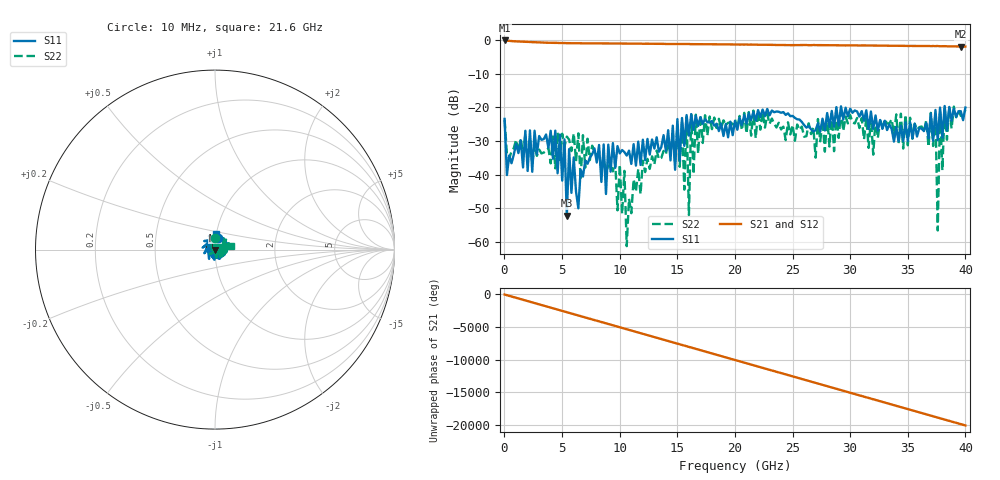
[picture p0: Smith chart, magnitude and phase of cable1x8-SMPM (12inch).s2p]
!Keysight Technologies,N5225A,MY51451228,A.10.40.14
!Date: Monday, November 23, 2020 09:38:04
!Correction: S22(Full 2 Port(2,4))
!S42(Full 2 Port(2,4))
!S24(Full 2 Port(2,4))
!S44(Full 2 Port(2,4))
!S2P File: Measurements: S22, S42, S24, S44:
# Hz S  dB  R 50
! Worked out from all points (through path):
!   201 points, 10 MHz to 40 GHz, reference 50 ohm
!   highest |S21| = -0.07 dB at 10 MHz (marker M1); lowest = -1.9 dB at 39.6 GHz (marker M2)
!   lowest |S11| = -52.3 dB at 5.409 GHz (marker M3), VSWR 1.00, Z = 50.1 - j0.208 ohm
!   |S11| at or under -10 dB: start of sweep to end of sweep
!   |S22| runs from -61.3 to -19.8 dB; largest |S21 - S12| = 0.0086
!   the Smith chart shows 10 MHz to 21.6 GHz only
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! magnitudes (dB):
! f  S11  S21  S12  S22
! 10 MHz  -23.4  -0.1  -0.1  -23.7
! 5.209 GHz  -29.5  -0.9  -0.9  -31.6
! 5.409 GHz  -52.3  -0.9  -0.9  -28.7
! 5.609 GHz  -32.4  -0.9  -0.9  -29.6
! 6.808 GHz  -40.6  -0.9  -0.9  -28.3
! 10.41 GHz  -33.3  -1.0  -1.0  -38.9
! 10.61 GHz  -34.3  -1.0  -1.0  -61.3
! 13.41 GHz  -33.2  -1.1  -1.1  -35.5
! 15.41 GHz  -23.2  -1.1  -1.1  -23.9
! 15.61 GHz  -31.5  -1.1  -1.1  -44.5
! 15.81 GHz  -22.3  -1.1  -1.1  -22.8
! 16.01 GHz  -28.4  -1.1  -1.1  -52.1
! 16.21 GHz  -22.0  -1.2  -1.1  -22.1
! 16.41 GHz  -26.7  -1.2  -1.1  -39.9
! 20 GHz  -24.1  -1.3  -1.3  -23.6
! 26.8 GHz  -27.2  -1.4  -1.5  -26.0
! 33.4 GHz  -25.0  -1.6  -1.7  -24.8
! 37.4 GHz  -20.8  -1.7  -1.8  -21.6
! 37.6 GHz  -29.7  -1.7  -1.8  -56.6
! 37.8 GHz  -20.0  -1.8  -1.8  -20.8
! 39.6 GHz  -21.1  -1.9  -1.9  -22.5
! 40 GHz  -20.0  -1.9  -2.0  -20.7
